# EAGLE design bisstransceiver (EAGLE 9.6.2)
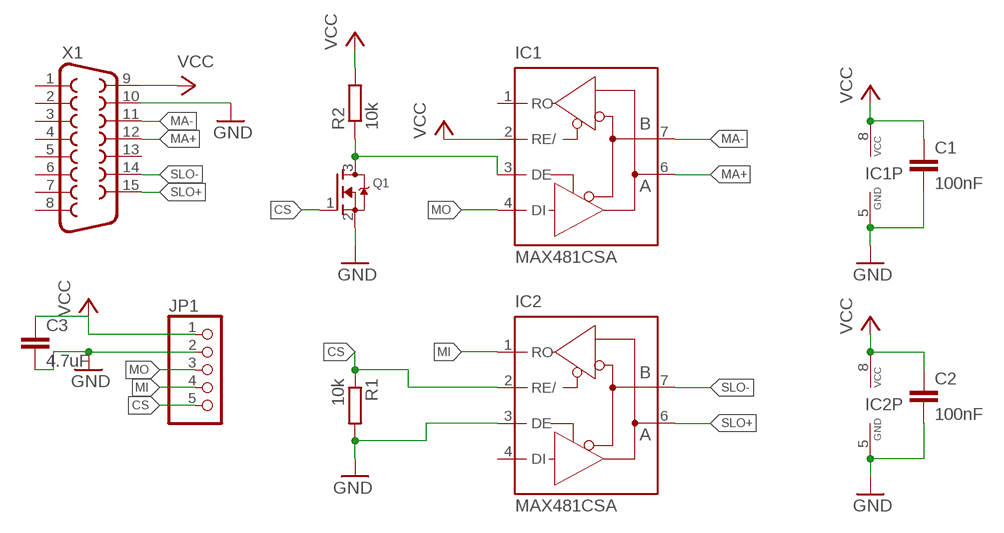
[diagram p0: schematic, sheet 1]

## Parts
C1  100nF  C-EUC0603  [C0603]
C2  100nF  C-EUC0603  [C0603]
C3  4.7uF  C-EUC0603  [C0603]
IC1  MAX481CSA  [SO08]
IC2  MAX481CSA  [SO08]
JP1  PINHD-1X5/90  [1X05/90]
Q1  MOSFET-NREFLOW  [SOT23]
R1  10k  R-EU_R0603  [R0603]
R2  10k  R-EU_R0603  [R0603]
X1  F15HP  [F15HP]

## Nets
CS: IC2.2(RE/) JP1.5 Q1.1(G) R1.1
GND: C1.2 C2.2 C3.2 IC1.5(GND) IC2.3(DE) IC2.5(GND) JP1.2 Q1.2(S) R1.2 X1.10
MA+: IC1.6(A) X1.12
MA-: IC1.7(B) X1.11
MI: IC2.1(RO) JP1.4
MO: IC1.4(DI) JP1.3
N$1: IC1.3(DE) Q1.3(D) R2.1
SLO+: IC2.6(A) X1.15
SLO-: IC2.7(B) X1.14
VCC: C1.1 C2.1 C3.1 IC1.2(RE/) IC1.8(VCC) IC2.8(VCC) JP1.1 R2.2 X1.9
Unconnected: IC1.1(RO) IC2.4(DI) X1.1 X1.2 X1.3 X1.4 X1.5 X1.6 X1.7 X1.8 X1.13

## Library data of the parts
C1-C3 = resistor:C-EU: CAPACITOR, European symbol
IC1 IC2 = maxim:MAX481CSA: RS485 TRANSEIVER; MF: MAXIM; MPN: MAX481CSA; OC_FARNELL: unknown; OC_NEWARK: 90C3817
JP1 = pinhead:PINHD-1X5: PIN HEADER
Q1 = adafruit:MOSFET-N: N-Channel Mosfet 2N7002E - 60V 260mA SOT23 [Digikey: 2N7002ET1GOSTR-ND] - REEL BSH103 - 30V 850mA SOT23 [Digikey: 568-5013-1-ND]
R1 R2 = resistor:R-EU_: RESISTOR, European symbol
X1 = con-subd:F15: SUB-D; OC_FARNELL: unknown; OC_NEWARK: unknown

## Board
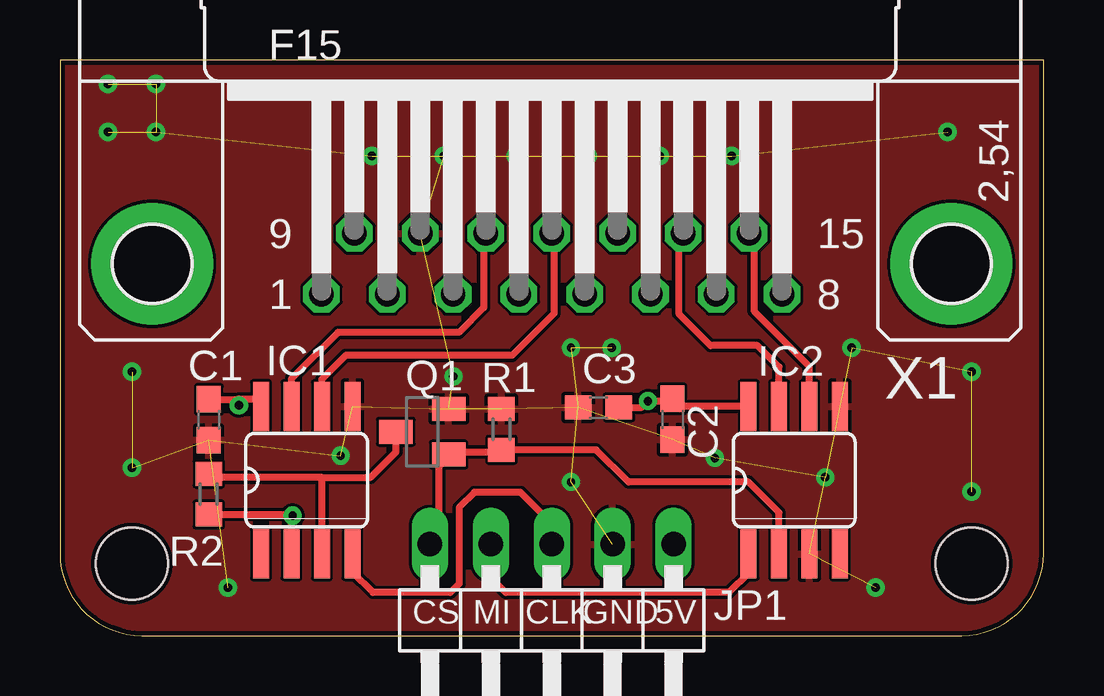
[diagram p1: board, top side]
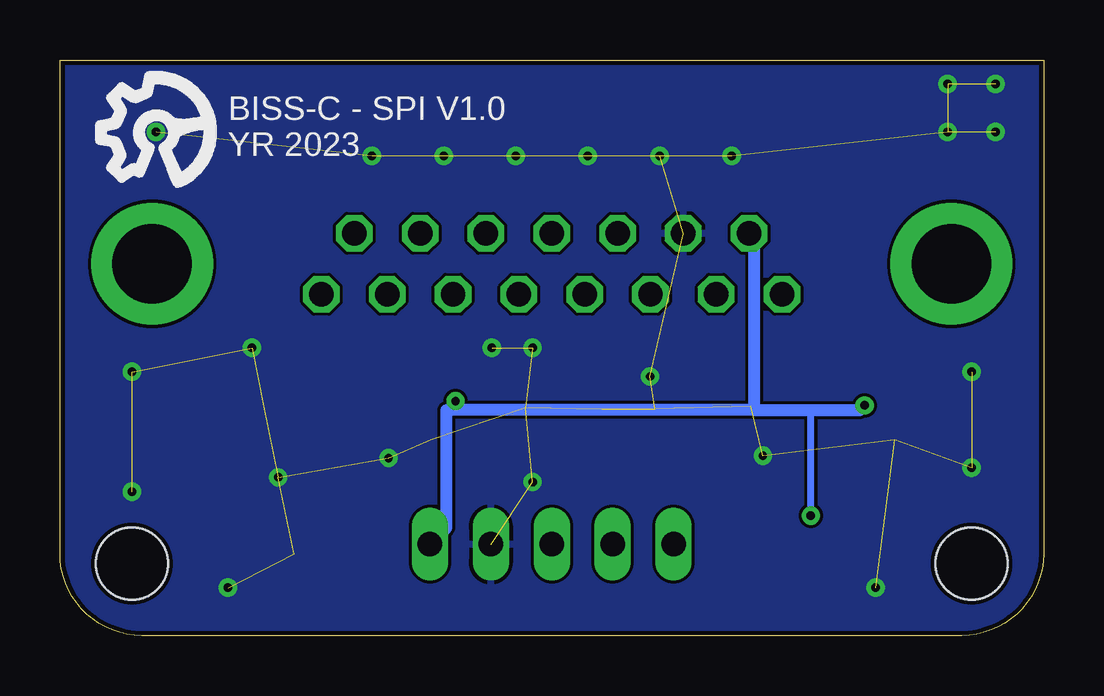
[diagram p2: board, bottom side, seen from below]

Size 41 x 24 mm. Coordinates in mm from the lower left corner, seen from the top.
Outline: 0,24 0,3.41 arc90 3.41,0 37.59,0 arc90 41,3.41 41,24 0,24
Copper layers (1*16): Top 0.035mm / dielectric 1.5mm / Bottom 0.035mm
Design rules "jlcpcb *": minimum track width 5mil, minimum drill 0.3mm, track to track 5mil, track to pad 5mil, pad to pad 5mil, via to via 5mil, smd to smd 5mil, copper to edge 0.2mm, drill to drill 8mil, minimum pad ring 10mil, minimum via ring 8mil, stop-mask expansion 4mil, vias tented up to drill 0.35mm, thermal gap 6mil
Holes 3 mm at 3,3 38,3

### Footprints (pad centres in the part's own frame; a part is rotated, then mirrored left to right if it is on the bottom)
C0603 = smd 1.1 x 1: 1 -0.85,0; 2 0.85,0
SO08 = smd 0.66 x 2.032: 1 -1.905,-3.073; 2 -0.635,-3.073; 3 0.635,-3.073; 4 1.905,-3.073; 5 1.905,3.073; 6 0.635,3.073; 7 -0.635,3.073; 8 -1.905,3.073
1X05/90 = drill 1.016 long: 1 -5.08,-3.81; 2 -2.54,-3.81; 3 0,-3.81; 4 2.54,-3.81; 5 5.08,-3.81
SOT23 = smd 1 x 1.4: 1 -0.95,-1.1; 2 0.95,-1.1; 3 0,1.1
R0603 = smd 1 x 1.1: 1 -0.85,0; 2 0.85,0
F15HP = drill 1.016 octagon: 1 -9.601,-1.27; 2 -6.858,-1.27; 3 -4.115,-1.27; 4 -1.372,-1.27; 5 1.372,-1.27; 6 4.115,-1.27; 7 6.858,-1.27; 8 9.601,-1.27; 9 -8.23,1.27; 10 -5.486,1.27; 11 -2.743,1.27; 12 0,1.27; 13 2.743,1.27; 14 5.486,1.27; 15 8.23,1.27 | drill 3.302 pad 5.08: G1 -16.662,0; G2 16.662,0

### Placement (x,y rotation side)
C1  6.2,9 270 top
C2  25.53,9.02 270 top
C3  22.45,9.51 180 top
IC1  10.29,6.48 0 top
IC2  30.61,6.48 0 top
JP1  20.5,0 180 top
Q1  15.1,8.5 90 top
R1  18.4,8.6 90 top
R2  6.2,5.9 270 top
X1  20.5,15.5 0 top

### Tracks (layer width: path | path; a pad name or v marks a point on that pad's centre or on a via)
CS
  Top 0.3: Q1.1 16.3,7.65 16.4,7.65 | 16.4,7.65 18.3,7.65 R1.1 22.35,7.75 23.7,6.4 28.7,6.4 29.97,5.13 IC2.2 | JP1.5 15.8,4.19 15.8,7.05 16.4,7.65
GND  (via drill 0.35)  (34 unrouted)
  other vias: 2,23 2,21 4,21 4,23 3,11 3,7 38,6 37,21 38,11 27.3,7.4 21.3,6.4 33,12 16.4,10.8 7,2 34,2 31.9,6.6 21.3,12 23,12 13,20 16,20 19,20 22,20 25,20 28,20 11.7,7.5
  pour Top: 0.13,26.1 0.13,-0.77 41.3,-0.77 41.3,26.1
  pour Bottom: 0.13,26.1 0.13,-0.47 41.15,-0.47 41.15,26.1
MA+
  Top 0.3: IC1.6 10.92,10.69 11.91,11.68 18.85,11.68 20.6,13.43 20.6,16.67 X1.12
MA-
  Top 0.3: IC1.7 9.65,10.71 11.58,12.64 16.63,12.64 17.66,13.67 17.66,16.67 X1.11
MI
  Top 0.3: JP1.4 17.96,2.41 18.57,1.8 27.89,1.8 28.7,2.6 IC2.1
MO
  Top 0.3: JP1.3 20.5,4.67 19.2,5.97 17.27,5.97 16.64,5.33 16.64,2.16 16.27,1.79 13.04,1.79 12.19,2.64 IC1.4
N$1
  Top 0.3: Q1.3 14,7.65 12.95,6.6 10.9,6.6 | IC1.3 10.92,6.58 10.9,6.6 | R2.1 6.35,6.6 10.9,6.6
SLO+
  Top 0.3: IC2.6 31.22,9.58 31.22,11.25 28.93,13.54 28.93,16.57 X1.15
SLO-
  Top 0.3: IC2.7 29.97,11.2 29.08,12.09 27.12,12.09 25.79,13.43 25.79,16.57 X1.14
VCC  (via drill 0.35)
  Top 0.3: IC1.8 8.06,9.87 7.46,9.87 v7.46,9.6 7.46,9.79 7.4,9.85 C1.1 | IC2.8 25.84,9.55 25.61,9.78 | 25.61,9.78 C2.1 | 25.61,9.78 v24.51,9.78 24.25,9.51 C3.1 | IC1.2 9.65,4.95 | 9.65,4.95 v9.7,5 | R2.2 9.55,5.05 9.65,4.95
  Bottom 0.3: 24.89,9.4 v24.51,9.78 | v9.7,5 9.7,9.4
  Bottom 0.5: X1.9 12.07,16.57 12.07,9.4 | v7.46,9.6 7.66,9.4 9.7,9.4 12.07,9.4 | 12.07,9.4 24.89,9.4 24.89,4.5 JP1.1

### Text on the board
tPlace: CS | MI | CLK | GND | 5V
bPlace: BISS-C - SPI V1.0 / YR 2023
